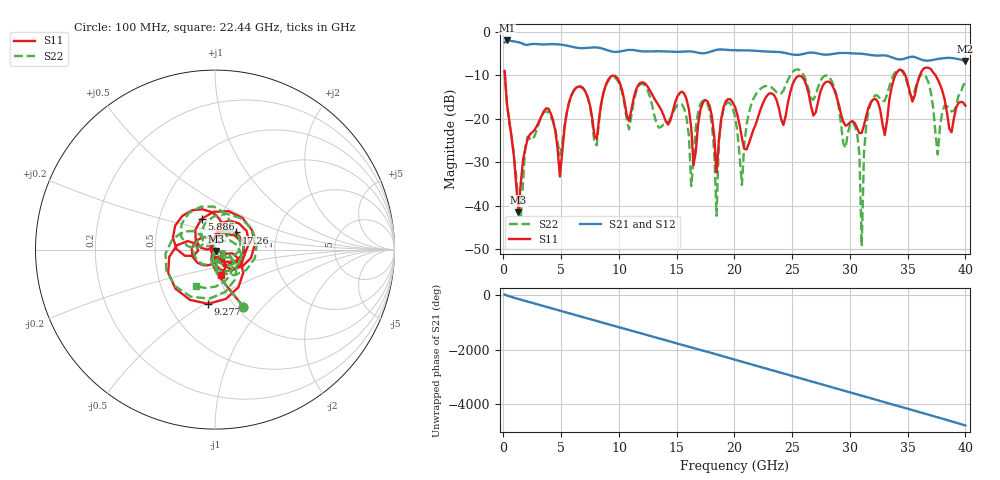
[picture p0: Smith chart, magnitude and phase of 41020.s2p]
!Agilent Technologies,N5230A,US43500312,A.07.50.67
!Agilent N5230A: A.07.50.67
!Date: Friday, June 16, 2023 12:48:05
!Correction: S11(Full 2 Port(1,2))
!S21(Full 2 Port(1,2))
!S12(Full 2 Port(1,2))
!S22(Full 2 Port(1,2))
!S2P File: Measurements: S11, S21, S12, S22:
# Hz S  dB  R 50
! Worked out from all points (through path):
!   201 points, 100 MHz to 40 GHz, reference 50 ohm
!   highest |S21| = -2.01 dB at 299.5 MHz (marker M1); lowest = -6.8 dB at 40 GHz (marker M2)
!   lowest |S11| = -41.5 dB at 1.297 GHz (marker M3), VSWR 1.02, Z = 50.4 - j0.76 ohm
!   |S11| at or under -10 dB: 126.5 MHz to 33.95 GHz (33.82 GHz wide, 199 % of centre); 34.8 GHz to 36.06 GHz (1.267 GHz wide, 3.58 % of centre); 37.41 GHz to end of sweep
!   |S22| runs from -49.3 to -8.6 dB; largest |S21 - S12| = 0.0028
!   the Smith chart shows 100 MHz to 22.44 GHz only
!   S11 on the Smith chart (normalised r, x): 100 MHz: 1.08, -0.78; 5.886 GHz: 0.81, +0.29; 9.277 GHz: 0.78, -0.52; 17.26 GHz: 1.24, +0.24; 22.44 GHz: 1.02, -0.30
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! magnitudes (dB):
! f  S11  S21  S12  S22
! 100 MHz  -9.0  -2.4  -2.4  -9.0
! 299.5 MHz  -16.5  -2.0  -2.0  -16.5
! 1.297 GHz  -41.5  -2.4  -2.4  -39.1
! 5.886 GHz  -14.6  -3.4  -3.4  -14.7
! 6.883 GHz  -13.0  -3.8  -3.8  -12.9
! 9.277 GHz  -10.3  -4.5  -4.5  -10.6
! 13.47 GHz  -17.0  -4.5  -4.5  -22.1
! 15.46 GHz  -13.8  -4.6  -4.6  -16.7
! 16.26 GHz  -22.0  -4.5  -4.5  -35.5
! 17.26 GHz  -16.4  -5.0  -5.0  -15.9
! 18.45 GHz  -32.3  -4.2  -4.2  -42.3
! 18.85 GHz  -20.1  -4.1  -4.1  -20.3
! 20.05 GHz  -17.3  -4.3  -4.3  -19.5
! 20.65 GHz  -24.5  -4.3  -4.3  -35.2
! 22.44 GHz  -16.6  -4.5  -4.5  -12.8
! 26.83 GHz  -19.3  -4.8  -4.8  -15.7
! 30.42 GHz  -21.0  -5.0  -5.0  -21.7
! 31.02 GHz  -23.3  -5.1  -5.1  -49.3
! 31.62 GHz  -17.4  -5.3  -5.3  -18.0
! 33.42 GHz  -15.6  -5.7  -5.7  -12.6
! 37.61 GHz  -11.0  -6.3  -6.3  -28.2
! 40 GHz  -17.0  -6.8  -6.8  -11.4
